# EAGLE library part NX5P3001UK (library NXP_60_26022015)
Bidirectional high-side power switch for charger and USB-OTG combined applications The NX5P3001 is an advanced bidirectional power switch and ESD-protection device for combined USB-OTG and charger port applications. It includes undervoltage lockout, overvoltage lockout and overtemperature protection circuits designed to automatically isolate the power switch terminals when a fault condition occurs. The device features two power switch input/output terminals (VBUSI and VBUSO), an open-drain acknowledge output (ACK), an enable input which includes logic level translation (EN) and low capacitance Transient Voltage Suppression (TVS) type ESD-clamps for USB data and ID pins. When EN is set HIGH the device enters a low-power mode, disabling all protection circuits. When used in combined charger and USB-OTG applications the 30 V tolerant VBUSI switch terminal is used as the supply and switch input when charging, for USB-OTG the VBUSO switch terminal is used as the supply and switch input. Designed for operation from 3.2 V to 6.35 V, it is used in battery charging and power domain isolation applications to reduce power dissipation and extend battery life. AAL Eindhoven MK
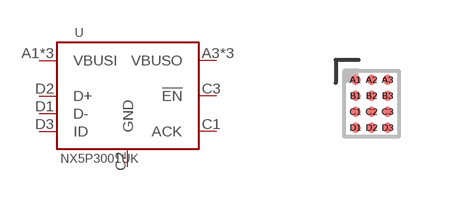
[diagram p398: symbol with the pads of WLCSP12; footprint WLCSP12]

Designator prefix U

## NX5P3001UK  [WLCSP12]
A1  VBUSI  pwr
A2  VBUSI  pwr
A3  VBUSO  pwr
B1  VBUSI  pwr
B2  VBUSO  pwr
B3  VBUSO  pwr
C1  ACK  out
C2  GND  pwr
C3  !EN  in
D1  D-  pas
D2  D+  pas
D3  ID  pas

## Footprint WLCSP12 (pad centres in mm)
smd 0.25 x 0.25: A1 -0.4,0.6; A2 0,0.6; A3 0.4,0.6; B1 -0.4,0.2; B2 0,0.2; B3 0.4,0.2; C1 -0.4,-0.2; C2 0,-0.2; C3 0.4,-0.2; D1 -0.4,-0.6; D2 0,-0.6; D3 0.4,-0.6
